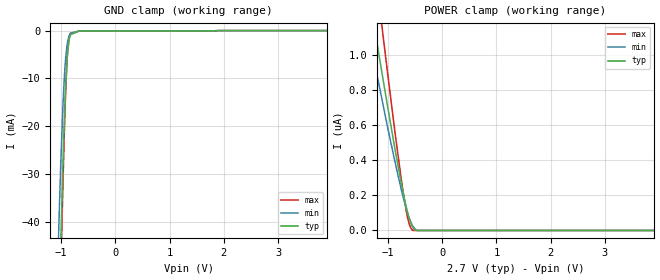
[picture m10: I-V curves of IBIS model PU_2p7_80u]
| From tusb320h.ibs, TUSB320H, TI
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|   Model
[Model]   PU_2p7_80u
Model_type   Input
Vinl = 0.81
Vinh = 1.89
|   typ   min   max
C_comp   0.475pF   0.451pF   0.489pF
[Voltage Range]   2.7   2.699   2.701
[Temperature Range]   27   105   -40
[Power Clamp Reference]   2.7   2.699   2.701
[GND Clamp Reference]   0   0   0
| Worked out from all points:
|   GND clamp passes 1 mA (typ) near -0.83 V on its own axis
[GND Clamp]
|   Voltage   I(typ)   I(min)   I(max)
-2.7V     -997.9mA   -935.7mA   -1.04A
-1.056V   -67.18mA   -46.42mA   -75.63mA
-1.04V    -59.47mA   -39.93mA   -67.26mA
-1.007V   -44.7mA    -27.99mA   -51.01mA
-966.6mV  -27.96mA   -15.65mA   -32.13mA
-942.3mV  -19.29mA   -10.04mA   -22.03mA
-918mV    -12.11mA   -5.957mA   -13.4mA
-893.7mV  -6.755mA   -3.293mA   -6.885mA
-877.5mV  -4.279mA   -2.155mA   -3.955mA
-828.9mV  -883.4uA   -583.2uA   -549.9uA
-666.9mV  -82.65uA   -76.14uA   -93.62uA
5.4V      0A         0A         0A
[POWER Clamp]
|   Voltage   I(typ)   I(min)   I(max)
-2.7V     3.977uA    3.304uA    5.388uA
-1.469V   1.576uA    1.306uA    2.096uA
-1.274V   1.206uA    999.7nA    1.586uA
-1.242V   1.145uA    949.1nA    1.502uA
-1.185V   1.038uA    861.2nA    1.354uA
-1.056V   797.1nA    663nA      1.022uA
-845.1mV  420nA      355.2nA    499.4nA
-666.9mV  138.9nA    128.9nA    117.6nA
-602.1mV  62.18nA    66.08nA    31.23nA
-537.3mV  15.04nA    22.98nA    0A
-464.4mV  0A         0A         0A
5.4V      0A         0A         0A
